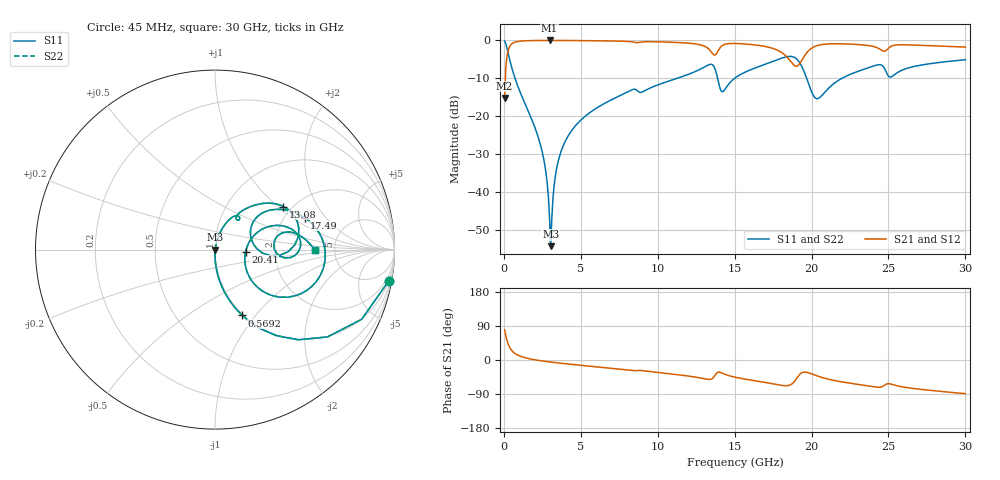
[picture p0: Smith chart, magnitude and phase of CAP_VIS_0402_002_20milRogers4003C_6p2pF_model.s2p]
! S-parameter model data by Modelithics Inc.  support@modelithics.com  813-866-6335  Tampa FL USA
! S-Parameter data specifications:
! Substrate: 20-mil Rogers 4003C, substrate thickness, H=0.508mm, Dielectric constant, Er=3.75
! PCB Mounting Pad Footprint: Pad width, PadW=0.50mm , Pad length, PadL=0.50mm , Pad gap, PadG (edge-to-edge)=0.40mm , Reference planes=1.4mm apart
! Created Wed Nov 18 12:48:53 2015
# hz S ma R 50
! 2 Port Network Data from SP1.SP block
! freq  magS11  angS11  magS21  angS21  magS12  angS12  magS22  angS22
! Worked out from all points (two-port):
!   401 points, 45 MHz to 30 GHz, reference 50 ohm
!   highest |S21| = -0.02 dB at 2.966 GHz (marker M1); lowest = -15.2 dB at 45 MHz (marker M2)
!   |S21| within 3 dB of the highest: 256.7 MHz to 13.48 GHz (13.22 GHz wide, 193 % of centre); 19.74 GHz to end of sweep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
!   lowest |S11| = -54.2 dB at 3.041 GHz (marker M3), VSWR 1.00, Z = 50.2 - j0.0173 ohm
!   |S11| at or under -10 dB: 721.9 MHz to 11.25 GHz (10.53 GHz wide, 176 % of centre); 13.89 GHz to 15 GHz (1.106 GHz wide, 7.66 % of centre); 19.68 GHz to 21.97 GHz (2.291 GHz wide, 11 % of centre)
!   |S22| runs from -54.2 to -0.1 dB; largest |S21 - S12| = 0
!   S11 on the Smith chart (normalised r, x): 45 MHz: 1, -11; 569.2 MHz: 0.99, -0.86; 13.08 GHz: 1.81, +1.09; 17.49 GHz: 2.54, +1.26; 20.41 GHz: 1.41, -0.04; 30 GHz: 3.50, -0.03
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4.5e7  0.9848 -10.1  0.1738 79.9  0.1738 79.9  0.9848 -10.1
2.696625e8  0.6841 -47.3  0.7289 42.7  0.7289 42.7  0.6841 -47.3
5.692125e8  0.3967 -67.5  0.9171 22.4  0.9171 22.4  0.3967 -67.5
2.366512e9  0.04267 -89.5  0.9973 -1.8  0.9973 -1.8  0.04267 -89.5
2.666062e9  0.02231 -88.8  0.9979 -3.5  0.9979 -3.5  0.02231 -88.8
2.965612e9  0.004622 -70.6  0.998 -5.1  0.998 -5.1  0.004622 -70.6
3.0405e9  0.00194 -5.1  0.998 -5.4  0.998 -5.4  0.00194 -5.1
3.414938e9  0.01986 76.8  0.9976 -7.2  0.9976 -7.2  0.01986 76.8
3.714488e9  0.03434 77.8  0.9971 -8.6  0.9971 -8.6  0.03434 77.8
5.062462e9  0.09149 74.1  0.9931 -14.3  0.9931 -14.3  0.09149 74.1
1.007992e10  0.2623 55.1  0.957 -33.2  0.957 -33.2  0.2623 55.1
1.307542e10  0.4506 32.2  0.8317 -49.8  0.8317 -49.8  0.4506 32.2
1.389919e10  0.3103 -6.4  0.712 -32.7  0.712 -32.7  0.3103 -6.4
1.427362e10  0.2145 22.9  0.8719 -36.1  0.8719 -36.1  0.2145 22.9
1.50225e10  0.3193 37.9  0.9104 -45.3  0.9104 -45.3  0.3193 37.9
1.749379e10  0.53 19.7  0.783 -63.0  0.783 -63.0  0.53 19.7
1.899154e10  0.5774 -20.8  0.4571 -50.9  0.4571 -50.9  0.5774 -20.8
2.003996e10  0.2018 -31.2  0.7984 -37.2  0.7984 -37.2  0.2018 -31.2
2.04144e10  0.1707 -4.5  0.8596 -42.7  0.8596 -42.7  0.1707 -4.5
2.408389e10  0.4635 11.3  0.8244 -70.9  0.8244 -70.9  0.4635 11.3
2.505742e10  0.3307 0.6  0.8054 -62.6  0.8054 -62.6  0.3307 0.6
3e10  0.5559 -0.3  0.8164 -88.9  0.8164 -88.9  0.5559 -0.3
